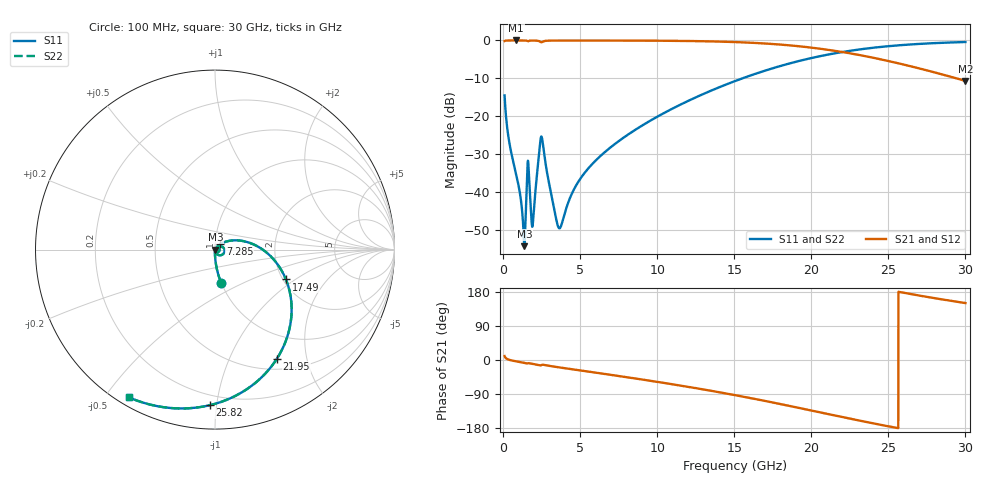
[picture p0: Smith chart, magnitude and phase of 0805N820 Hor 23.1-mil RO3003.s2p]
# GHz S MA R 50
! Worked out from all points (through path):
!   3201 points, 100 MHz to 30 GHz, reference 50 ohm
!   highest |S21| = -0.01 dB at 847.5 MHz (marker M1); lowest = -10.7 dB at 30 GHz (marker M2)
!   group delay of S21, straight-line fit = 20.2 ps
!   lowest |S11| = -54.3 dB at 1.38 GHz (marker M3), VSWR 1.00, Z = 50.2 - j0.0818 ohm
!   |S11| at or under -10 dB: start of sweep to 15.54 GHz
!   |S22| runs from -54.3 to -0.4 dB; largest |S21 - S12| = 0
!   S11 on the Smith chart (normalised r, x): 100 MHz: 1.00, -0.38; 7.285 GHz: 1.06, +0.07; 17.49 GHz: 2.07, -0.84; 21.95 GHz: 0.64, -1.52; 25.82 GHz: 0.14, -0.96; 30 GHz: 0.03, -0.57
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0.1  0.1881 -79.6  0.9818 10.3  0.9818 10.3  0.1881 -79.6
0.4083438  0.04458 -89.0  0.9985 0.4  0.9985 0.4  0.04458 -89.0
0.8475  0.01715 -91.2  0.9991 -3.6  0.9991 -3.6  0.01715 -91.2
1.099781  0.009463 -89.8  0.999 -5.4  0.999 -5.4  0.009463 -89.8
1.286656  0.004171 -78.8  0.9987 -6.7  0.9987 -6.7  0.004171 -78.8
1.380094  0.001923 -25.1  0.9981 -7.4  0.9981 -7.4  0.001923 -25.1
1.632375  0.0246 -26.8  0.9766 -8.3  0.9766 -8.3  0.0246 -26.8
1.847281  0.004179 -38.0  0.9962 -9.8  0.9962 -9.8  0.004179 -38.0
1.959406  0.004472 27.5  0.9964 -10.7  0.9964 -10.7  0.004472 27.5
2.333156  0.03218 36.7  0.9792 -14.0  0.9792 -14.0  0.03218 36.7
2.482656  0.05395 -11.3  0.946 -13.4  0.946 -13.4  0.05395 -11.3
3.631937  0.003322 -17.9  0.9965 -19.4  0.9965 -19.4  0.003322 -17.9
5.089563  0.01573 52.3  0.997 -28.0  0.997 -28.0  0.01573 52.3
7.285344  0.0434 45.3  0.9959 -40.9  0.9959 -40.9  0.0434 45.3
10.06978  0.1 30.0  0.9912 -58.1  0.9912 -58.1  0.1 30.0
15.05  0.2906 -3.7  0.9514 -92.7  0.9514 -92.7  0.2906 -3.7
17.48872  0.4285 -22.8  0.8972 -112.0  0.8972 -112.0  0.4285 -22.8
20.03956  0.5874 -44.2  0.802 -133.6  0.802 -133.6  0.5874 -44.2
21.94569  0.6994 -60.5  0.7067 -149.9  0.7067 -149.9  0.6994 -60.5
25.01978  0.8399 -85.6  0.5339 -175.1  0.5339 -175.1  0.8399 -85.6
25.82334  0.8668 -91.8  0.4895 178.7  0.4895 178.7  0.8668 -91.8
30  0.9529 -120.2  0.2924 150.3  0.2924 150.3  0.9529 -120.2
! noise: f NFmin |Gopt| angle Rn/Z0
0.1  0.0004704  0.8713  0.6428  0.0007875
3.417  0.008561  0.7727  18.31  0.007495
6.743  0.01037  0.6597  35.49  0.005307
10.06  0.01396  0.6371  51.69  0.005942
13.39  0.01808  0.6376  66.87  0.006691
16.7  0.02302  0.6524  80.98  0.007523
20.03  0.02932  0.6787  94.3  0.008505
23.35  0.03778  0.7148  107.1  0.009709
26.67  0.04989  0.7594  119.7  0.0112
30  0.06832  0.8095  132.3  0.01288
